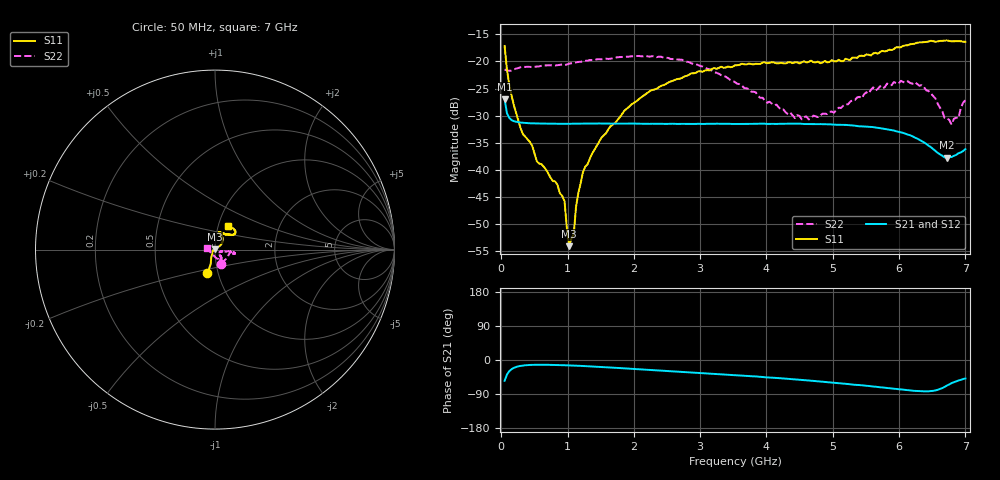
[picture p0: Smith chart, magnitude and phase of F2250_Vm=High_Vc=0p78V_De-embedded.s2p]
! Integrated Device Technology
! Corporate Headquarters
! 6024 Silver Creek Valley Road
! San Jose, CA 95138  USA
! Phone:  1-408-284-8200
! Toll Free:  1-800-223-1366
! Webpage:  http://www.idt.com/
! Timing and RF Division
! 515 Groton Road, Suite 102
! Westford, MA 01886-6024
! Device:  F2250
! Description: Voltage Variable RF Attenuator
! Frequency:  50.0 -  6000.00 MHz
! Package:  3x3 mm Thin QFN Plastic Package: 16 pin
! Ports:  2 RF, 3 DC
!  Pin  1  = GND
!  Pin  2  = NC
!  Pin  3  = RF1  = Port 1
!  Pin  4  = NC
!  Pin  5  = GND
!  Pin  6  = GND
!  Pin  7  = GND
!  Pin  8  = GND
!  Pin  9  = NC
!  Pin 10  = RF2  = Port 2
!  Pin 11  = NC
!  Pin 12  = GND
!  Pin 13  = GND
!  Pin 14  = VCNTRL
!  Pin 15  = VDD
!  Pin 16  = VMODE
! Vcntrl:  0.780 Volts
! Vmode:  +3.300 Volts
! Vdd:  +3.30  Volts
! Current:  1.301 mA
! Data:  The device was measured on a the F2250 evaluation board which has
!  individual transmission lines to the RF pins.  Data was collected
!  using a calibrated network analyzer.  The evaluation board was
!  de-embedded using a TRL calibration technique.
!  The reference plane is the edge of the package pin.
! Misc:  SN 10
!  Action Tracker AT0258
! Date Measured:  2014-11-26
! Date:  2015-10-15  MJV
! Note:
!  Integrated Device Technology supplies this data as a sample of measured
!  data at the package pin for this product.  Your particular data for this
!  product may vary.
!  Data was taken at 25 degrees C.
!  Integrated Device Technology reserves the right to change this data at anytime.
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# GHz S dB R 50
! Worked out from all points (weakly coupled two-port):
!   201 points, 50 MHz to 7 GHz, reference 50 ohm
!   highest |S21| = -26.99 dB at 50 MHz (marker M1); lowest = -37.7 dB at 6.722 GHz (marker M2)
!   lowest |S11| = -54.1 dB at 1.023 GHz (marker M3), VSWR 1.00, Z = 49.9 + j0.148 ohm
!   |S11| at or under -10 dB: start of sweep to end of sweep
!   |S22| runs from -31.6 to -19.0 dB; largest |S21 - S12| = 0.0001
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0.05  -17.14 -107.8  -26.99 -54.7  -26.99 -54.7  -21.47 -66.5
0.1195  -24.20 -110.9  -30.40 -29.6  -30.40 -29.6  -21.71 -21.3
0.29325  -32.40 -125.1  -31.27 -15.5  -31.28 -15.5  -21.04 -10.9
0.467  -35.58 -143.7  -31.41 -12.9  -31.39 -12.8  -21.02 -7.7
0.5365  -38.43 -151.5  -31.43 -12.6  -31.43 -12.6  -20.94 -8.3
0.8145  -42.13 171.0  -31.48 -13.1  -31.49 -13.1  -20.75 -10.2
0.9535  -45.74 172.8  -31.50 -13.8  -31.50 -13.9  -20.67 -11.4
1.023  -54.06 131.6  -31.49 -14.3  -31.48 -14.3  -20.39 -11.5
1.0925  -51.95 68.4  -31.48 -14.7  -31.47 -14.7  -20.31 -11.7
1.12725  -46.78 49.1  -31.47 -15.0  -31.47 -15.0  -20.18 -12.2
1.2315  -40.41 35.1  -31.46 -15.8  -31.46 -15.8  -19.95 -13.3
1.6485  -31.91 39.1  -31.46 -19.8  -31.47 -19.8  -19.49 -12.9
2.37825  -24.74 45.7  -31.49 -27.5  -31.49 -27.5  -19.11 -10.8
3.525  -20.71 71.2  -31.52 -40.0  -31.52 -40.0  -23.82 -9.6
4.4285  -20.17 74.3  -31.48 -51.2  -31.48 -51.2  -30.45 -24.9
4.7065  -20.13 71.7  -31.55 -55.1  -31.54 -55.1  -29.98 -34.4
5.85325  -17.83 40.3  -32.60 -74.5  -32.58 -74.6  -24.40 -54.0
6.33975  -16.50 40.5  -34.67 -82.4  -34.67 -82.5  -24.37 -67.7
6.722  -16.13 49.1  -37.72 -67.3  -37.73 -67.3  -30.42 -120.3
6.7915  -16.28 51.0  -37.62 -61.0  -37.59 -61.1  -31.64 -139.6
6.89575  -16.25 56.2  -36.93 -54.0  -36.92 -54.0  -30.46 -169.1
7  -16.38 62.1  -36.17 -48.8  -36.18 -48.7  -27.15 171.5
